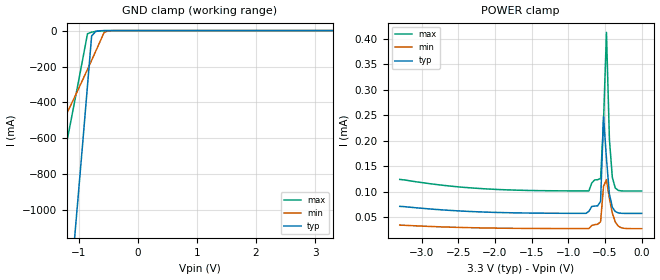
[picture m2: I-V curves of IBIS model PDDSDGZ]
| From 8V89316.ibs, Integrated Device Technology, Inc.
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|   Model PDDSDGZ
[Model]  PDDSDGZ
Model_type Input
Polarity   Non-Inverting
Vinl =   0.8000V
Vinh =   2.0000V
C_comp   2.6812pF   2.6701pF   2.6826pF
[Temperature Range]   25.0000   0.1250k   -40.0000
[Voltage Range]   3.3000V   3.0000V   3.6000V
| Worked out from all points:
|   GND clamp passes 1 mA (typ) near -0.64 V on its own axis
[GND_clamp]
|Voltage   I(typ)   I(min)   I(max)
-3.3V     -8.473A    -1.702A    -3.67A
-2.25V    -5.322A    -1.128A    -2.26A
-2.18V    -5.094A    -1.087A    -2.158A
-1.55V    -2.941A    -695.2mA   -1.195A
-1.48V    -2.689A    -649.4mA   -1.083A
-1.06V    -1.126A    -365mA     -383.4mA
-850mV    -308.3mA   -216.3mA   -17.65mA
-780mV    -30.2mA    -165.7mA   -8.739mA
-710mV    -4.257mA   -114.6mA   -4.589mA
-570mV    -195.9uA   -10.81mA   -435.6uA
-500mV    -58.31uA   -1.732mA   -98.01uA
3.3V      57.9uA     29.96uA    101.7uA
[POWER_clamp]
|Voltage   I(typ)   I(min)   I(max)
-3.3V     71.8uA     35.04uA    124.4uA
-2.16V    60.67uA    29.52uA    106.2uA
-720mV    61.92uA    28.24uA    101.9uA
-680mV    71.62uA    34.23uA    117.6uA
-560mV    81.4uA     41.85uA    126.2uA
-520mV    247.4uA    111uA      238.4uA
-480mV    165.3uA    124.1uA    412.1uA
-440mV    95.84uA    86.88uA    203.4uA
-400mV    70.17uA    58.44uA    128.3uA
-360mV    61.63uA    41.31uA    107.7uA
-320mV    58.98uA    33.21uA    103uA
0V        57.91uA    28.11uA    101.8uA
